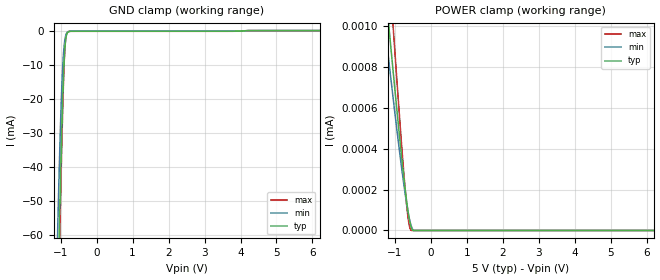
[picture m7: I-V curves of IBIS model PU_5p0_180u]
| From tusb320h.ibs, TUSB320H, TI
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|   Model
[Model]   PU_5p0_180u
Model_type   Input
Vinl = 1.5
Vinh = 3.5
|   typ   min   max
C_comp   0.475pF   0.451pF   0.489pF
[Voltage Range]   5   4.999   5.001
[Temperature Range]   27   105   -40
[Power Clamp Reference]   5   4.999   5.001
[GND Clamp Reference]   0   0   0
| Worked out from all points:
|   GND clamp passes 1 mA (typ) near -0.83 V on its own axis
[GND Clamp]
|   Voltage   I(typ)   I(min)   I(max)
-5V       -2.345A    -2.242A    -2.422A
-1.085V   -81.56mA   -58.86mA   -91.13mA
-1.04V    -59.74mA   -40.17mA   -67.54mA
-1.025V   -52.78mA   -34.44mA   -59.92mA
-995mV    -39.5mA    -24mA      -45.2mA
-965mV    -27.4mA    -15.29mA   -31.47mA
-935mV    -17.02mA   -8.721mA   -19.31mA
-905mV    -9.067mA   -4.448mA   -9.683mA
-890mV    -6.19mA    -3.075mA   -6.196mA
-860mV    -2.572mA   -1.431mA   -2.097mA
-800mV    -453.5uA   -376.6uA   -321.8uA
10V       0A         0A         0A
[POWER Clamp]
|   Voltage   I(typ)   I(min)   I(max)
-5V       8.523uA    1.593A     11.61uA
-1.91V    2.427uA    87.48uA    3.265uA
-1.25V    1.158uA    959.6nA    1.521uA
-1.145V   960.8nA    797.1nA    1.249uA
-1.04V    766.4nA    637.3nA    979.9nA
-830mV    392.3nA    332.2nA    461.8nA
-695mV    176.2nA    158.2nA    166.7nA
-650mV    114.5nA    108.4nA    88.13nA
-605mV    62.54nA    65.62nA    31.31nA
-530mV    8.341nA    15.64nA    0A
-485mV    0A         0A         0A
10V       0A         0A         0A
